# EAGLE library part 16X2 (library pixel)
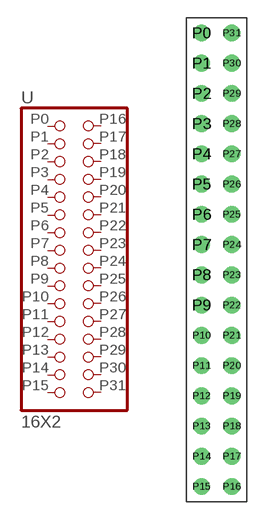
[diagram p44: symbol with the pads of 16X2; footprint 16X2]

Designator prefix -

## 16X2  [16X2]
P0  P0  pas
P1  P1  pas
P2  P2  pas
P3  P3  pas
P4  P4  pas
P5  P5  pas
P6  P6  pas
P7  P7  pas
P8  P8  pas
P9  P9  pas
P10  P10  pas
P11  P11  pas
P12  P12  pas
P13  P13  pas
P14  P14  pas
P15  P15  pas
P16  P16  pas
P17  P17  pas
P18  P18  pas
P19  P19  pas
P20  P20  pas
P21  P21  pas
P22  P22  pas
P23  P23  pas
P24  P24  pas
P25  P25  pas
P26  P26  pas
P27  P27  pas
P28  P28  pas
P29  P29  pas
P30  P30  pas
P31  P31  pas

## Footprint 16X2 (pad centres in mm)
drill 0.9 pad 1.27: P0 -1.27,19.05; P1 -1.27,16.51; P2 -1.27,13.97; P3 -1.27,11.43; P4 -1.27,8.89; P5 -1.27,6.35; P6 -1.27,3.81; P7 -1.27,1.27; P8 -1.27,-1.27; P9 -1.27,-3.81; P10 -1.27,-6.35; P11 -1.27,-8.89; P12 -1.27,-11.43; P13 -1.27,-13.97; P14 -1.27,-16.51; P15 -1.27,-19.05; P16 1.27,-19.05; P17 1.27,-16.51; P18 1.27,-13.97; P19 1.27,-11.43; P20 1.27,-8.89; P21 1.27,-6.35; P22 1.27,-3.81; P23 1.27,-1.27; P24 1.27,1.27; P25 1.27,3.81; P26 1.27,6.35; P27 1.27,8.89; P28 1.27,11.43; P29 1.27,13.97; P30 1.27,16.51; P31 1.27,19.05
